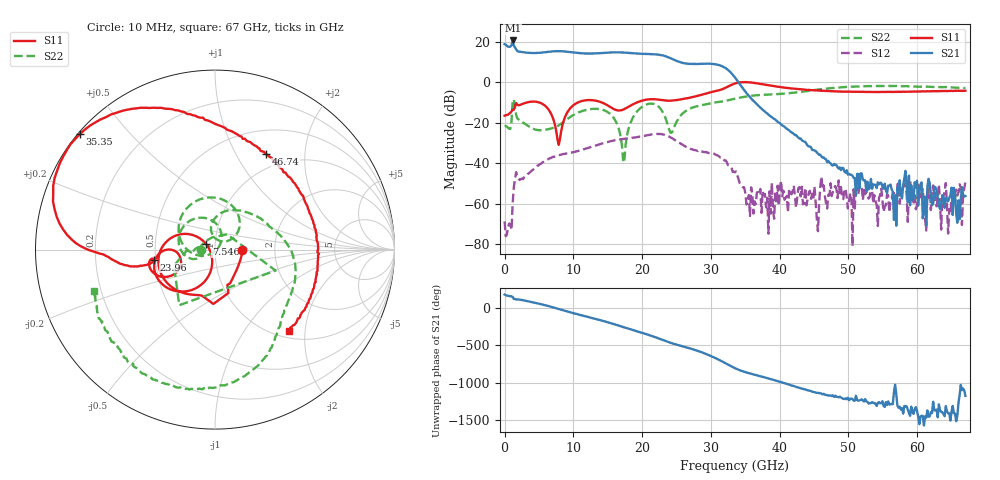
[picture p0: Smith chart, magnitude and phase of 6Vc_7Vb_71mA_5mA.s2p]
! MARKI MICROWAVE INC.
! Date:  05/05/2020
! Model Number:  APM-7099CH
! Description:  2-port Small Signal S-parameter data for APM-7099CH
! Frequency Range:  10 MHz to 67 GHz
! Port Configuration:  PORT 1: Input
!  PORT 2: Output
! Bias Condition: Vc = +6V, Vb = +7V
! APM-7099CH s2p files are only valid for small signal conditions (below -5 dBm input power)
!S2P File: Measurements: Mag<S11> Ang<S11>, Mag<S21> Ang<S21>, Mag<S12> Ang<S12>, Mag<S22> Ang<S22>!row 1
# Hz S  dB  R 50
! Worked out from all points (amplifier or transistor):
!   401 points, 10 MHz to 67 GHz, reference 50 ohm
!   highest |S21| = 20.5 dB at 1.182 GHz (marker M1)
!   |S21| within 3 dB of that: start of sweep to 482.7 MHz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
!   unconditionally stable (mu >= 1): start of sweep to end of sweep
!   at 11.06 GHz: K = 4.11, MAG = 14.9 dB, |S12| = -33.7 dB
!   at 33.51 GHz: K = 8.50, MAG = 11.1 dB, |S12| = -44.6 dB
!   at 67 GHz: K = 30061.66, MAG = -51.3 dB, |S12| = -49.4 dB
!   S11 on the Smith chart (normalised r, x): 10 MHz: 1.35, -0.00; 7.546 GHz: 0.91, +0.05; 23.96 GHz: 0.49, -0.06; 35.35 GHz: 0.01, +0.37; 46.74 GHz: 0.80, +1.34; 67 GHz: 1.13, -1.64
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1e7  -16.61 -0.4  18.69 178.4  -68.86 2.5  -21.99 -177.6
1.182325e9  -13.74 -65.8  20.54 144.9  -59.81 78.6  -8.94 -19.1
1.68475e9  -10.37 -91.7  16.31 112.4  -44.49 -82.4  -16.12 -178.4
4.866775e9  -9.91 -170.6  14.39 58.8  -41.35 -176.6  -23.77 179.5
7.546375e9  -24.82 148.4  15.24 -6.3  -36.48 118.0  -22.02 -157.4
9.3886e9  -13.65 -111.1  14.87 -55.6  -35.11 77.6  -17.63 -156.3
1.123082e10  -9.38 -140.7  14.21 -100.4  -33.53 43.7  -14.40 -179.3
1.47478e10  -11.07 -179.4  14.47 174.1  -29.81 -29.9  -14.37 111.7
1.60876e10  -13.67 -173.9  14.67 136.9  -28.73 -61.7  -18.92 74.8
1.759488e10  -13.04 -152.4  14.51 93.6  -27.96 -99.0  -31.26 -128.3
2.027448e10  -8.95 -156.9  13.89 17.5  -26.62 -165.9  -11.64 136.1
2.245165e10  -8.72 -170.7  13.50 -50.9  -25.65 127.6  -12.34 59.3
2.395892e10  -9.24 -170.6  12.03 -102.0  -26.98 75.0  -23.76 44.2
2.6806e10  -7.84 -167.5  8.97 -179.0  -32.42 6.9  -13.38 77.7
2.931812e10  -5.63 -171.1  9.09 101.7  -34.52 -45.6  -10.97 44.9
3.132782e10  -3.92 -177.9  8.23 16.7  -37.22 -107.0  -9.71 25.0
3.3505e10  -0.71 165.8  2.21 -88.1  -44.61 152.1  -8.17 8.2
3.534722e10  -0.08 139.4  -6.12 -149.8  -59.44 90.1  -7.02 -7.5
4.472582e10  -4.01 72.0  -33.50 -42.2  -55.21 -64.4  -4.11 -59.3
4.673552e10  -4.39 61.7  -38.10 -87.5  -59.82 -52.8  -3.25 -69.4
5.594665e10  -4.86 8.7  -51.25 146.0  -64.35 -156.6  -1.96 -116.3
6.7e10  -4.29 -47.8  -56.34 -98.5  -49.38 24.4  -2.97 -161.3
